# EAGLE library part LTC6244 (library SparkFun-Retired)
Low-noise, high-speed rail-to-rail CMOS op-amp Not in catalog
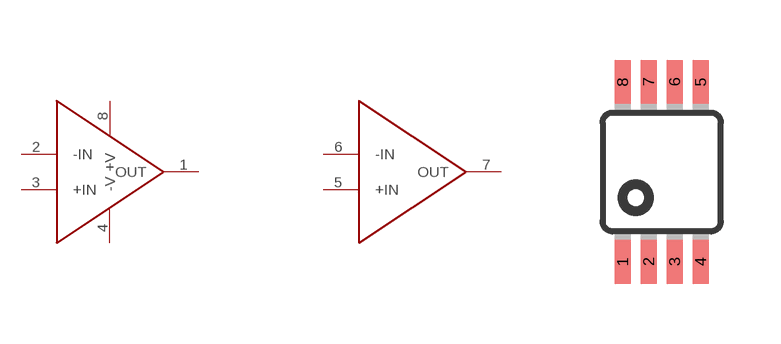
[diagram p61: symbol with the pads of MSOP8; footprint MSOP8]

Designator prefix -; gates G1=LTC6244 G2=LTC6244_2

## LTC6244  [MSOP8]
1  G1:OUT
2  G1:-IN
3  G1:+IN
4  G1:-V
5  G2:+IN
6  G2:-IN
7  G2:OUT
8  G1:+V

## Footprint MSOP8 (pad centres in mm)
8M, 8-Lead, 0.118" Wide, Miniature Small Outline Package MSOP 8M-Package doc1097.pdf
smd 0.4 x 1.1: 1 -0.975,-2.25; 2 -0.325,-2.25; 3 0.325,-2.25; 4 0.975,-2.25; 5 0.975,2.25; 6 0.325,2.25; 7 -0.325,2.25; 8 -0.975,2.25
